| TEXAS INSTRUMENTS INCORPORATED
| Standard Linear and Logic Group
| IBIS Model of SN74ALVCHR16601
| 18-BIT UNIVERSAL BUS TRANSCEIVER WITH 3-STATE OUTPUTS
| This file contains package information for the following:
|  TSSOP 56-pin (DGG) package as [Component] ALVCHR16601_DGG
|  TVSOP 56-pin (DGV) package as [Component] ALVCHR16601_DGV
|  SSOP 56-pin (DL) package as [Component] ALVCHR16601_DL
| This device can be powered at the following Vccs:
|  1.8 volt Vcc
|  2.5 volt Vcc
|  3.3 volt Vcc
| This file provides unique models under the [Model Selector] for each Vcc.
| For operation at a specific Vcc, select the appropriate model after each
| [Model Selector] keyword.
[IBIS Ver]   3.2
[Comment char]  |_char
[File Name]   sn74alvchr16601.ibs
[File Rev]   1.1 | b_die
[Date]   May 19, 2004
[Source]   Data created from TI-SPICE simulations at TI-SLL.
[Notes]   The following is an IBIS list for the ALVCHR16601.
   Please contact sllibis@ti.com with questions and
   comments concerning SLL IBIS models.
   This IBIS model is created from a BA (back annotated netlist)
   - FILE REV HISTORY
   - 1.1 Release IBIS file on 06/07/04
   - Due to presence of bus hold at input, GND-clamp curves
   have non-monotonic warnings.
   - Non-monotonic data in pullup/pulldown data due to resistor.
[Disclaimer] Property of Texas Instruments Incorporated.  Unauthorized
   reproduction and/or distribution is strictly prohibited.
   This product is protected under copyright law.
   Created  2001, (C) Copyright  2001, Texas Instruments
   Incorporated, All Rights Reserved
   UNLESS THERE IS A SIGNED, WRITTEN AGREEMENT TO THE
   CONTRARY, TEXAS INSTRUMENTS (TI) IS PROVIDING THE IBIS
   MODELS  AND WITHOUT ANY WARRANTY, EXPRESSED OR
   IMPLIED.  TI assumes no liability for:
   1) the accuracy of the IBIS models provided to your
   company;
   2) the proper functioning of these IBIS Models in your
   design or for any resulting applications; or
   3) infringement of patents, copyrights or intellectual
   property rights resulting from your use of these IBIS
   models.
   TI provides IBIS Models as a service to our customers.
   You and your company shall not distribute, sell or give
   these models to anyone else without prior written
   permission from TI.
   TI reserves the right to make changes to our products or
   to discontinue any semiconductor product or service
   without notice, and advises our customers to obtain the
   latest version of relevant information to verify, before
   placing orders, that the information being relied on is
   current.
   Please be aware that your receipt and use of the IBIS
   information provided shall serve as acceptance of these
   terms and conditions.  If you do not accept these terms,
   you should return or destroy the IBIS models and any
   other accompanying information immediately.
| Component ALVCHR16601_DGG 56-pin TSSOP
[Component]   ALVCHR16601_DGG
[Manufacturer]   Texas Instruments, Inc.
[Package]
|   typ   min   max
R_pkg   4.500e-02   3.500e-02   6.200e-02
L_pkg   3.324e-09   2.403e-09   5.094e-09
C_pkg   5.640e-13   3.410e-13   9.140e-13
[Pin]   signal_name   model_name   R_pin   L_pin   C_pin
1   NOEAB   ALVCHR16601_NOE   6.200e-02   5.094e-09   8.560e-13
2   LEAB   ALVCHR16601_LE   6.100e-02   4.621e-09   9.020e-13
3   A1   ALVCHR16601_IO   6.000e-02   4.316e-09   8.020e-13
4   GND   GND   5.900e-02   3.968e-09   6.980e-13
5   A2   ALVCHR16601_IO   5.700e-02   3.716e-09   6.490e-13
6   A3   ALVCHR16601_IO   4.200e-02   3.517e-09   6.520e-13
7   VCC   POWER   4.100e-02   3.160e-09   5.700e-13
8   A4   ALVCHR16601_IO   3.900e-02   2.981e-09   4.820e-13
9   A5   ALVCHR16601_IO   3.900e-02   2.809e-09   4.470e-13
10   A6   ALVCHR16601_IO   3.800e-02   2.715e-09   4.090e-13
11   GND   GND   4.100e-02   2.675e-09   3.910e-13
12   A7   ALVCHR16601_IO   3.900e-02   2.536e-09   3.660e-13
13   A8   ALVCHR16601_IO   3.900e-02   2.457e-09   3.480e-13
14   A9   ALVCHR16601_IO   3.800e-02   2.411e-09   3.530e-13
15   A10   ALVCHR16601_IO   3.900e-02   2.456e-09   3.550e-13
16   A11   ALVCHR16601_IO   3.900e-02   2.471e-09   3.490e-13
17   A12   ALVCHR16601_IO   4.000e-02   2.580e-09   3.700e-13
18   GND   GND   3.800e-02   2.651e-09   3.890e-13
19   A13   ALVCHR16601_IO   3.800e-02   2.739e-09   4.110e-13
20   A14   ALVCHR16601_IO   3.900e-02   2.838e-09   4.490e-13
21   A15   ALVCHR16601_IO   3.800e-02   2.988e-09   4.840e-13
22   VCC   POWER   3.800e-02   3.105e-09   5.640e-13
23   A16   ALVCHR16601_IO   4.000e-02   3.427e-09   6.380e-13
24   A17   ALVCHR16601_IO   5.600e-02   3.654e-09   6.410e-13
25   GND   GND   5.700e-02   3.932e-09   7.000e-13
26   A18   ALVCHR16601_IO   5.800e-02   4.257e-09   8.060e-13
27   NOEBA   ALVCHR16601_NOE   5.700e-02   4.580e-09   9.140e-13
28   LEBA   ALVCHR16601_LE   5.900e-02   5.038e-09   8.610e-13
29   NCLKENBA   ALVCHR16601_CEN   6.000e-02   5.058e-09   8.580e-13
30   CLKBA   ALVCHR16601_CLK   5.600e-02   4.543e-09   9.040e-13
31   B18   ALVCHR16601_IO   5.700e-02   4.240e-09   8.030e-13
32   GND   GND   5.700e-02   3.929e-09   7.000e-13
33   B17   ALVCHR16601_IO   5.600e-02   3.616e-09   6.370e-13
34   B16   ALVCHR16601_IO   3.700e-02   3.368e-09   6.400e-13
35   VCC   POWER   3.600e-02   3.024e-09   5.630e-13
36   B15   ALVCHR16601_IO   3.500e-02   2.876e-09   4.740e-13
37   B14   ALVCHR16601_IO   3.500e-02   2.745e-09   4.440e-13
38   B13   ALVCHR16601_IO   3.700e-02   2.683e-09   4.050e-13
39   GND   GND   3.800e-02   2.603e-09   3.820e-13
40   B12   ALVCHR16601_IO   3.800e-02   2.510e-09   3.620e-13
41   B11   ALVCHR16601_IO   3.600e-02   2.412e-09   3.410e-13
42   B10   ALVCHR16601_IO   3.800e-02   2.416e-09   3.490e-13
43   B9   ALVCHR16601_IO   3.700e-02   2.403e-09   3.490e-13
44   B8   ALVCHR16601_IO   3.700e-02   2.429e-09   3.410e-13
45   B7   ALVCHR16601_IO   3.600e-02   2.482e-09   3.580e-13
46   GND   GND   3.700e-02   2.615e-09   3.810e-13
47   B6   ALVCHR16601_IO   3.500e-02   2.669e-09   4.020e-13
48   B5   ALVCHR16601_IO   3.600e-02   2.763e-09   4.420e-13
49   B4   ALVCHR16601_IO   3.600e-02   2.942e-09   4.780e-13
50   VCC   POWER   3.500e-02   3.053e-09   5.640e-13
51   B3   ALVCHR16601_IO   3.600e-02   3.409e-09   6.410e-13
52   B2   ALVCHR16601_IO   5.800e-02   3.698e-09   6.410e-13
53   GND   GND   5.900e-02   3.975e-09   6.970e-13
54   B1   ALVCHR16601_IO   6.100e-02   4.327e-09   8.020e-13
55   CLKAB   ALVCHR16601_CLK   6.100e-02   4.624e-09   9.050e-13
56   NCLKENAB   ALVCHR16601_CEN   6.000e-02   5.063e-09   8.580e-13
| Component ALVCHR16601_DGV 56-pin TVSOP
[Component]   ALVCHR16601_DGV
[Manufacturer]   Texas Instruments, Inc.
[Package]
|   typ   min   max
R_pkg   6.300e-02   5.000e-02   8.600e-02
L_pkg   2.945e-09   2.392e-09   3.938e-09
C_pkg   3.910e-13   2.710e-13   5.880e-13
[Pin]   signal_name   model_name   R_pin   L_pin   C_pin
1   NOEAB   ALVCHR16601_NOE   6.800e-02   3.933e-09   5.880e-13
2   LEAB   ALVCHR16601_LE   6.800e-02   3.569e-09   5.860e-13
3   A1   ALVCHR16601_IO   7.600e-02   3.464e-09   5.150e-13
4   GND   GND   8.600e-02   3.451e-09   4.580e-13
5   A2   ALVCHR16601_IO   8.200e-02   3.278e-09   4.260e-13
6   A3   ALVCHR16601_IO   7.700e-02   3.143e-09   3.870e-13
7   VCC   POWER   6.900e-02   2.971e-09   4.010e-13
8   A4   ALVCHR16601_IO   5.000e-02   2.787e-09   3.790e-13
9   A5   ALVCHR16601_IO   5.100e-02   2.686e-09   3.200e-13
10   A6   ALVCHR16601_IO   5.200e-02   2.607e-09   3.160e-13
11   GND   GND   5.300e-02   2.497e-09   2.970e-13
12   A7   ALVCHR16601_IO   5.400e-02   2.438e-09   2.920e-13
13   A8   ALVCHR16601_IO   5.500e-02   2.412e-09   2.860e-13
14   A9   ALVCHR16601_IO   5.500e-02   2.400e-09   2.730e-13
15   A10   ALVCHR16601_IO   5.500e-02   2.402e-09   2.730e-13
16   A11   ALVCHR16601_IO   5.400e-02   2.398e-09   2.840e-13
17   A12   ALVCHR16601_IO   5.400e-02   2.407e-09   2.890e-13
18   GND   GND   5.300e-02   2.448e-09   2.930e-13
19   A13   ALVCHR16601_IO   5.200e-02   2.548e-09   3.110e-13
20   A14   ALVCHR16601_IO   5.100e-02   2.623e-09   3.160e-13
21   A15   ALVCHR16601_IO   5.000e-02   2.725e-09   3.700e-13
22   VCC   POWER   6.500e-02   2.903e-09   3.940e-13
23   A16   ALVCHR16601_IO   7.300e-02   3.086e-09   3.870e-13
24   A17   ALVCHR16601_IO   8.200e-02   3.272e-09   4.280e-13
25   GND   GND   8.200e-02   3.394e-09   4.570e-13
26   A18   ALVCHR16601_IO   7.100e-02   3.374e-09   5.080e-13
27   NOEBA   ALVCHR16601_NOE   6.900e-02   3.572e-09   5.810e-13
28   LEBA   ALVCHR16601_LE   6.900e-02   3.937e-09   5.740e-13
29   NCLKENBA   ALVCHR16601_CEN   6.900e-02   3.923e-09   5.690e-13
30   CLKBA   ALVCHR16601_CLK   6.800e-02   3.546e-09   5.740e-13
31   B18   ALVCHR16601_IO   7.400e-02   3.422e-09   5.180e-13
32   GND   GND   8.100e-02   3.395e-09   4.680e-13
33   B17   ALVCHR16601_IO   8.000e-02   3.255e-09   4.310e-13
34   B16   ALVCHR16601_IO   7.100e-02   3.063e-09   3.860e-13
35   VCC   POWER   6.100e-02   2.878e-09   3.900e-13
36   B15   ALVCHR16601_IO   5.000e-02   2.709e-09   3.640e-13
37   B14   ALVCHR16601_IO   5.100e-02   2.607e-09   3.110e-13
38   B13   ALVCHR16601_IO   5.100e-02   2.532e-09   3.060e-13
39   GND   GND   5.300e-02   2.440e-09   2.890e-13
40   B12   ALVCHR16601_IO   5.300e-02   2.399e-09   2.860e-13
41   B11   ALVCHR16601_IO   5.400e-02   2.392e-09   2.820e-13
42   B10   ALVCHR16601_IO   5.500e-02   2.399e-09   2.710e-13
43   B9   ALVCHR16601_IO   5.500e-02   2.395e-09   2.710e-13
44   B8   ALVCHR16601_IO   5.500e-02   2.403e-09   2.830e-13
45   B7   ALVCHR16601_IO   5.400e-02   2.421e-09   2.880e-13
46   GND   GND   5.300e-02   2.472e-09   2.920e-13
47   B6   ALVCHR16601_IO   5.100e-02   2.569e-09   3.090e-13
48   B5   ALVCHR16601_IO   5.100e-02   2.636e-09   3.130e-13
49   B4   ALVCHR16601_IO   5.000e-02   2.739e-09   3.660e-13
50   VCC   POWER   6.500e-02   2.922e-09   3.900e-13
51   B3   ALVCHR16601_IO   7.200e-02   3.076e-09   3.840e-13
52   B2   ALVCHR16601_IO   8.100e-02   3.249e-09   4.300e-13
53   GND   GND   8.300e-02   3.400e-09   4.550e-13
54   B1   ALVCHR16601_IO   7.300e-02   3.421e-09   5.060e-13
55   CLKAB   ALVCHR16601_CLK   6.900e-02   3.579e-09   5.780e-13
56   NCLKENAB   ALVCHR16601_CEN   6.900e-02   3.938e-09   5.810e-13
| Component ALVCHR16601_DL 56-pin SSOP
[Component]   ALVCHR16601_DL
[Manufacturer]   Texas Instruments, Inc.
[Package]
|   typ   min   max
R_pkg   5.500e-02   4.800e-02   6.700e-02
L_pkg   6.539e-09   4.802e-09   9.746e-09
C_pkg   1.880e-13   7.600e-14   5.170e-13
[Pin]   signal_name   model_name   R_pin   L_pin   C_pin
1   NOEAB   ALVCHR16601_NOE   6.400e-02   9.646e-09   5.130e-13
2   LEAB   ALVCHR16601_LE   5.900e-02   8.723e-09   2.700e-13
3   A1   ALVCHR16601_IO   5.900e-02   8.139e-09   2.230e-13
4   GND   GND   5.600e-02   7.554e-09   2.010e-13
5   A2   ALVCHR16601_IO   5.400e-02   6.991e-09   1.950e-13
6   A3   ALVCHR16601_IO   5.300e-02   6.659e-09   2.020e-13
7   VCC   POWER   5.500e-02   6.321e-09   2.070e-13
8   A4   ALVCHR16601_IO   5.500e-02   5.942e-09   1.330e-13
9   A5   ALVCHR16601_IO   5.700e-02   5.767e-09   1.320e-13
10   A6   ALVCHR16601_IO   5.400e-02   5.459e-09   1.210e-13
11   GND   GND   5.100e-02   5.224e-09   1.400e-13
12   A7   ALVCHR16601_IO   4.800e-02   5.088e-09   1.260e-13
13   A8   ALVCHR16601_IO   5.000e-02   5.021e-09   9.600e-14
14   A9   ALVCHR16601_IO   5.100e-02   4.802e-09   7.600e-14
15   A10   ALVCHR16601_IO   5.100e-02   4.803e-09   7.600e-14
16   A11   ALVCHR16601_IO   5.000e-02   5.021e-09   9.600e-14
17   A12   ALVCHR16601_IO   4.800e-02   5.088e-09   1.260e-13
18   GND   GND   5.100e-02   5.224e-09   1.400e-13
19   A13   ALVCHR16601_IO   5.400e-02   5.459e-09   1.210e-13
20   A14   ALVCHR16601_IO   5.700e-02   5.768e-09   1.330e-13
21   A15   ALVCHR16601_IO   5.500e-02   5.942e-09   1.330e-13
22   VCC   POWER   5.500e-02   6.320e-09   2.060e-13
23   A16   ALVCHR16601_IO   5.300e-02   6.659e-09   2.030e-13
24   A17   ALVCHR16601_IO   5.400e-02   6.991e-09   1.960e-13
25   GND   GND   5.600e-02   7.554e-09   2.010e-13
26   A18   ALVCHR16601_IO   5.900e-02   8.139e-09   2.230e-13
27   NOEBA   ALVCHR16601_NOE   5.900e-02   8.727e-09   2.700e-13
28   LEBA   ALVCHR16601_LE   6.700e-02   9.746e-09   5.170e-13
29   NCLKENBA   ALVCHR16601_CEN   6.300e-02   9.630e-09   5.110e-13
30   CLKBA   ALVCHR16601_CLK   6.000e-02   8.751e-09   2.710e-13
31   B18   ALVCHR16601_IO   6.000e-02   8.184e-09   2.250e-13
32   GND   GND   5.600e-02   7.543e-09   2.000e-13
33   B17   ALVCHR16601_IO   5.400e-02   7.005e-09   1.960e-13
34   B16   ALVCHR16601_IO   5.600e-02   6.714e-09   2.040e-13
35   VCC   POWER   5.800e-02   6.384e-09   2.080e-13
36   B15   ALVCHR16601_IO   5.700e-02   5.976e-09   1.340e-13
37   B14   ALVCHR16601_IO   5.700e-02   5.743e-09   1.300e-13
38   B13   ALVCHR16601_IO   5.400e-02   5.468e-09   1.190e-13
39   GND   GND   5.500e-02   5.328e-09   1.420e-13
40   B12   ALVCHR16601_IO   5.200e-02   5.189e-09   1.290e-13
41   B11   ALVCHR16601_IO   5.200e-02   5.053e-09   9.600e-14
42   B10   ALVCHR16601_IO   5.100e-02   4.825e-09   7.600e-14
43   B9   ALVCHR16601_IO   5.400e-02   4.896e-09   7.800e-14
44   B8   ALVCHR16601_IO   5.200e-02   5.093e-09   9.700e-14
45   B7   ALVCHR16601_IO   5.100e-02   5.179e-09   1.280e-13
46   GND   GND   5.400e-02   5.314e-09   1.420e-13
47   B6   ALVCHR16601_IO   5.500e-02   5.511e-09   1.210e-13
48   B5   ALVCHR16601_IO   5.700e-02   5.771e-09   1.310e-13
49   B4   ALVCHR16601_IO   5.600e-02   5.957e-09   1.330e-13
50   VCC   POWER   5.500e-02   6.320e-09   2.060e-13
51   B3   ALVCHR16601_IO   5.200e-02   6.621e-09   2.000e-13
52   B2   ALVCHR16601_IO   5.300e-02   6.973e-09   1.950e-13
53   GND   GND   5.700e-02   7.571e-09   2.020e-13
54   B1   ALVCHR16601_IO   5.700e-02   8.097e-09   2.220e-13
55   CLKAB   ALVCHR16601_CLK   5.900e-02   8.723e-09   2.710e-13
56   NCLKENAB   ALVCHR16601_CEN   6.100e-02   9.560e-09   5.090e-13
| Model ALVCHR16601_CEN
[Model Selector]   ALVCHR16601_CEN
ALVCHR16601_CEN_18   1.8 volt Vcc
ALVCHR16601_CEN_25   2.5 volt Vcc
ALVCHR16601_CEN_33   3.3 volt Vcc
| Model ALVCHR16601_CLK
[Model Selector]   ALVCHR16601_CLK
ALVCHR16601_CLK_18   1.8 volt Vcc
ALVCHR16601_CLK_25   2.5 volt Vcc
ALVCHR16601_CLK_33   3.3 volt Vcc
| Model ALVCHR16601_NOE
[Model Selector]   ALVCHR16601_NOE
ALVCHR16601_NOE_18   1.8 volt Vcc
ALVCHR16601_NOE_25   2.5 volt Vcc
ALVCHR16601_NOE_33   3.3 volt Vcc
| Model ALVCHR16601_LE
[Model Selector]   ALVCHR16601_LE
ALVCHR16601_LE_18   1.8 volt Vcc
ALVCHR16601_LE_25   2.5 volt Vcc
ALVCHR16601_LE_33   3.3 volt Vcc
| Model ALVCHR16601_IO
[Model Selector]   ALVCHR16601_IO
ALVCHR16601_IO_18   1.8 volt Vcc
ALVCHR16601_IO_25   2.5 volt Vcc
ALVCHR16601_IO_33   3.3 volt Vcc
| Models and submodels in the file (15): ALVCHR16601_CEN_18 (Input), ALVCHR16601_CEN_25 (Input), ALVCHR16601_CEN_33 (Input), ALVCHR16601_CLK_18 (Input), ALVCHR16601_CLK_25 (Input), ALVCHR16601_CLK_33 (Input), ALVCHR16601_NOE_18 (Input), ALVCHR16601_NOE_25 (Input), ALVCHR16601_NOE_33 (Input), ALVCHR16601_LE_18 (Input), ALVCHR16601_LE_25 (Input), ALVCHR16601_LE_33 (Input), ALVCHR16601_IO_18 (I/O), ALVCHR16601_IO_25 (I/O), ALVCHR16601_IO_33 (I/O)
